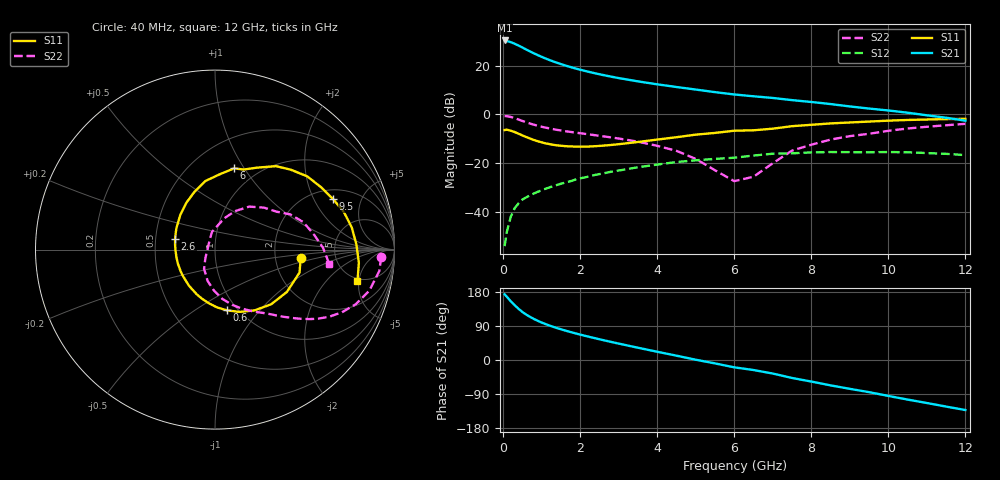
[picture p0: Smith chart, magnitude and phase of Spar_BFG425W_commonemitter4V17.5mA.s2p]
! Filename: 417bfg425.001
! BFG425W Field C1
! V1=8.378E-001V,V2=4.000E+000V, I1=2.095E-004A, I2=1.749E-002A
# GHz  S  MA  R 50
!  S11  S21  S12  S22
!Freq(GHz)  Mag  Ang  Mag  Ang  Mag  Ang  Mag  Ang
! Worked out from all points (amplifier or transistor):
!   44 points, 40 MHz to 12 GHz, reference 50 ohm
!   highest |S21| = 30.3 dB at 40 MHz (marker M1)
!   |S21| within 3 dB of that: start of sweep to 515 MHz
!   unconditionally stable (mu >= 1): start of sweep to 49.96 MHz; 1.445 GHz to end of sweep
!   at 700 MHz: K = 0.71, MSG = 29.5 dB, |S12| = -33.2 dB
!   at 2.4 GHz: K = 1.13, MAG = 18.6 dB, |S12| = -24.7 dB
!   at 12 GHz: K = 1.35, MAG = 3.5 dB, |S12| = -16.7 dB
!   S11 on the Smith chart (normalised r, x): 40 MHz: 2.80, -0.32; 600 MHz: 0.89, -0.69; 2.6 GHz: 0.63, +0.08; 6 GHz: 0.78, +0.90; 9.5 GHz: 2.50, +2.87; 12 GHz: 4.59, -4.79
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0.04  0.48 -5.3  32.9 173.4  0.002 45.0  0.927 -2.5
0.1  0.488 -15.2  31.98 166.6  0.004 74.2  0.923 -7.5
0.2  0.465 -30.4  30.41 154.9  0.008 71.8  0.89 -14.8
0.3  0.437 -44.1  28.21 144.6  0.012 69.0  0.842 -21.2
0.4  0.404 -56.9  25.9 135.3  0.015 66.0  0.789 -26.3
0.5  0.373 -68.6  23.63 126.8  0.018 63.2  0.738 -30.4
0.6  0.345 -78.8  21.48 119.8  0.02 61.6  0.692 -33.8
0.8  0.3 -97.0  17.93 108.3  0.024 59.0  0.617 -38.7
0.9  0.283 -104.8  16.48 103.4  0.026 58.1  0.587 -40.7
1  0.269 -112.3  15.2 98.9  0.028 57.4  0.561 -42.5
1.2  0.248 -125.8  13.11 91.1  0.032 56.2  0.519 -45.7
1.6  0.225 -149.5  10.19 78.1  0.04 53.7  0.457 -51.2
2.2  0.22 -178.4  7.562 62.0  0.053 48.8  0.394 -59.9
2.6  0.23 165.2  6.429 52.4  0.062 44.8  0.357 -66.2
3.5  0.273 135.2  4.772 32.4  0.083 33.9  0.277 -81.6
4.5  0.342 109.5  3.659 11.4  0.106 19.7  0.18 -103.1
6  0.465 76.8  2.571 -19.4  0.13 -4.5  0.043 149.2
6.5  0.474 70.2  2.36 -26.4  0.144 -7.5  0.053 127.4
8.5  0.656 38.5  1.635 -67.0  0.17 -44.5  0.306 51.5
9.5  0.716 23.1  1.323 -84.8  0.168 -61.3  0.402 31.7
10.5  0.772 9.2  1.088 -104.4  0.168 -80.0  0.516 17.2
12  0.813 -12.6  0.746 -132.1  0.147 -110.3  0.643 -7.4
